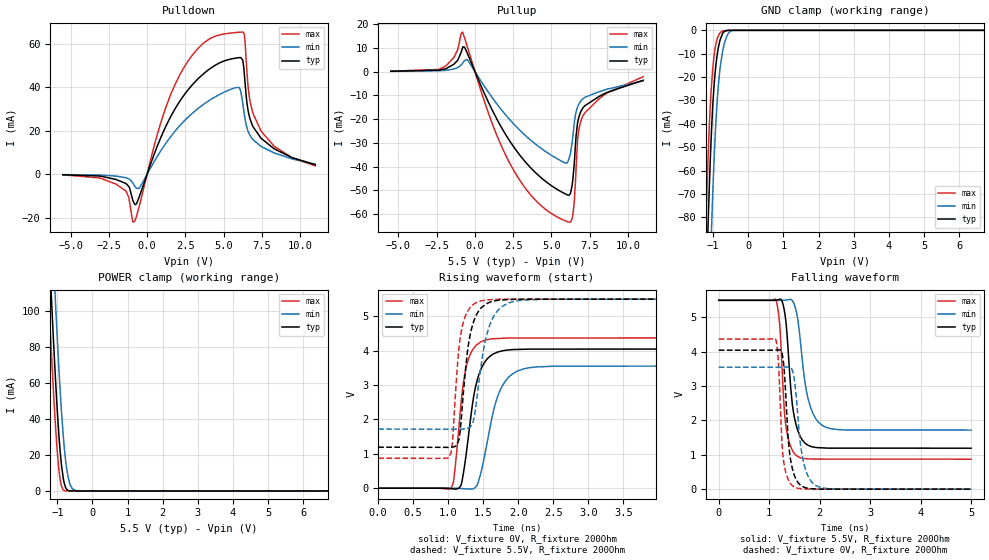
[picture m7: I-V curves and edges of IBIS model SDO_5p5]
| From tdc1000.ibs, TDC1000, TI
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|   Model
[Model]   SDO_5p5
Model_type   I/O
Polarity   Non-Inverting
Enable   Active-Low
Vinl = 1.65
Vinh = 3.85
Vmeas = 2.25
Vref = 0
Cref = 1pF
Rref = 100000
|   typ   min   max
C_comp   0.670pF   0.613pF   0.704pF
[Voltage Range]   5.5   5.499   5.501
[Temperature Range]   27   125   -40
[Pullup Reference]   5.5   5.499   5.501
[Pulldown Reference]   0   0   0
[Power Clamp Reference]   5.5   5.499   5.501
[GND Clamp Reference]   0   0   0
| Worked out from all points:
|   slope of the pulldown table from 0 to 0.825 V, typ, clamps not added: 52.8 ohm
|   slope of the pullup table from 0 to 0.825 V, typ, clamps not added: 68.1 ohm
|   GND clamp passes 1 mA (typ) near -0.72 V on its own axis
|   POWER clamp passes 1 mA (typ) near -0.74 V on its own axis
|   falling waveform, V_fixture 5.5V, R_fixture 200Ohm: 20-80 % time 159ps typ, 216ps min, 117ps max; typ from 5.5 V to 1.19 V
|   rising waveform, V_fixture 0V, R_fixture 200Ohm: 20-80 % time 183ps typ, 244ps min, 142ps max; typ from 0 V to 4.05 V
|   rising waveform, V_fixture 5.5V, R_fixture 200Ohm: 20-80 % time 146ps typ, 192ps min, 113ps max; typ from 1.19 V to 5.5 V
|   falling waveform, V_fixture 0V, R_fixture 200Ohm: 20-80 % time 122ps typ, 166ps min, 90.8ps max; typ from 4.05 V to 0 V
[Pulldown]
|   Voltage   I(typ)   I(min)   I(max)
-5.5V     -159.5uA   -111.1uA   -197.3uA
-2.018V   -2.354mA   -771.3uA   -4.488mA
-1.375V   -4.191mA   -1.551mA   -7.639mA
-896.5mV  -12.53mA   -4.359mA   -21.94mA
1.018V    18.82mA    12.1mA     26.35mA
2.321V    35.45mA    23.74mA    47.99mA
3.987V    47.87mA    33.59mA    61.79mA
6.116V    53.67mA    38.45mA    65.32mA
6.347V    47.19mA    28.17mA    64.54mA
6.71V     26.04mA    18.19mA    34.61mA
7.452V    16.63mA    12.87mA    19.92mA
11V       4.448mA    4.629mA    3.918mA
[GND Clamp]
|   Voltage   I(typ)   I(min)   I(max)
-5.5V     -2.812A    -2.859A    -2.771A
-1.21V    -116.3mA   -165.8mA   -85.32mA
-1.144V   -83.18mA   -131.3mA   -54.52mA
-1.095V   -60.96mA   -106.9mA   -36.38mA
-1.045V   -42.43mA   -84.13mA   -23.12mA
-962.5mV  -21.54mA   -51.78mA   -9.662mA
-863.5mV  -8.444mA   -25.81mA   -2.724mA
-797.5mV  -3.887mA   -15.56mA   -985.5uA
-731.5mV  -1.371mA   -8.982mA   -335.7uA
-583mV    -36.18uA   -1.672mA   -12.75uA
-368.5mV  -49.95nA   -10.8uA    0A
11V       0A         0A         0A
[Pullup]
|   Voltage   I(typ)   I(min)   I(max)
-5.5V     126.3uA    85.09uA    152.6uA
-1.887V   1.218mA    511.7uA    2.419mA
-814mV    9.921mA    3.459mA    16.59mA
1.166V    -16.67mA   -11.29mA   -22.47mA
2.552V    -31.83mA   -22.16mA   -41.75mA
4.235V    -44.13mA   -31.86mA   -55.84mA
6.165V    -51.95mA   -36.34mA   -63.33mA
6.396V    -45.57mA   -27.5mA    -60.43mA
6.512V    -36.89mA   -20.65mA   -52.82mA
6.726V    -20.93mA   -14.61mA   -27.58mA
7.056V    -15.29mA   -11.44mA   -18.58mA
11V       -3.655mA   -3.933mA   -2.15mA
[POWER Clamp]
|   Voltage   I(typ)   I(min)   I(max)
-5.5V     2.447A     2.527A     2.372A
-1.243V   140.2mA    188.7mA    107.4mA
-1.177V   111.5mA    158.6mA    80.61mA
-1.062V   65.64mA    108.8mA    39.2mA
-995.5mV  43.07mA    82.81mA    20.63mA
-929.5mV  24.57mA    59.3mA     7.823mA
-880mV    14.17mA    43.81mA    2.591mA
-797.5mV  3.942mA    23.23mA    191uA
-731.5mV  829.6uA    12.13mA    34.62uA
-665.5mV  103.2uA    5.44mA     7.356uA
-451mV    96.8nA     72.72uA    0A
11V       0A         0A         0A
[Ramp]
R_load = 200
|   typ   min   max
dV/dt_r   2.42832/1.83085e-10   2.13189/2.44228e-10   2.62284/1.41744e-10
dV/dt_f   2.58416/1.58879e-10   2.26726/2.16097e-10   2.77665/1.16684e-10
[Falling Waveform]
V_fixture = 5.5V
V_fixture_min = 5.499V
V_fixture_max = 5.501V
R_fixture = 200Ohm
C_fixture = 0F
|   Time   V(typ)   V(min)   V(max)
0s        5.5V       5.499V     5.501V
1.129ns   5.505V     5.498V     5.518V
1.207ns   5.528V     5.498V     4.799V
1.288ns   5.294V     5.502V     2.565V
1.335ns   4.817V     5.507V     1.793V
1.459ns   2.458V     5.487V     1.13V
1.564ns   1.718V     4.965V     951.9mV
1.774ns   1.274V     2.613V     884mV
2.061ns   1.202V     1.846V     875.4mV
5ns       1.193V     1.72V      873.2mV
[Rising Waveform]
V_fixture = 0V
V_fixture_min = 0V
V_fixture_max = 0V
R_fixture = 200Ohm
C_fixture = 0F
|   Time   V(typ)   V(min)   V(max)
0s        -5.038uV   998.1nV    -272.4nV
1.051ns   -14.6mV    645.7uV    35.31mV
1.092ns   -23.56mV   1.142mV    485.1mV
1.177ns   67.6mV     -8.1mV     2.345V
1.243ns   795.2mV    -16.07mV   3.395V
1.362ns   2.65V      -8.849mV   4.065V
1.466ns   3.458V     453.6mV    4.259V
1.693ns   3.948V     2.592V     4.352V
1.982ns   4.035V     3.403V     4.369V
5ns       4.047V     3.553V     4.371V
[Rising Waveform]
V_fixture = 5.5V
V_fixture_min = 5.499V
V_fixture_max = 5.501V
R_fixture = 200Ohm
C_fixture = 0F
|   Time   V(typ)   V(min)   V(max)
0s        1.193V     1.72V      873.2mV
1.016ns   1.188V     1.717V     910.8mV
1.062ns   1.199V     1.716V     1.387V
1.133ns   1.312V     1.716V     3.629V
1.187ns   2.06V      1.716V     4.571V
1.282ns   4.092V     1.751V     5.164V
1.399ns   5.023V     2.446V     5.397V
1.567ns   5.387V     4.592V     5.48V
1.864ns   5.486V     5.388V     5.498V
5ns       5.5V       5.499V     5.501V
[Falling Waveform]
|Gnd
V_fixture = 0V
V_fixture_min = 0V
V_fixture_max = 0V
R_fixture = 200Ohm
C_fixture = 0F
|   Time   V(typ)   V(min)   V(max)
0s        4.047V     3.553V     4.371V
1.129ns   4.052V     3.553V     4.358V
1.187ns   4.056V     3.553V     3.571V
1.247ns   3.98V      3.555V     1.511V
1.288ns   3.613V     3.556V     792.2mV
1.388ns   1.268V     3.554V     245.9mV
1.513ns   350.6mV    3.012V     51.24mV
1.669ns   71.99mV    857.7mV    7.639mV
1.919ns   7.11mV     111.2mV    573.1uV
5ns       5.112uV    -987.3nV   7.543uV
